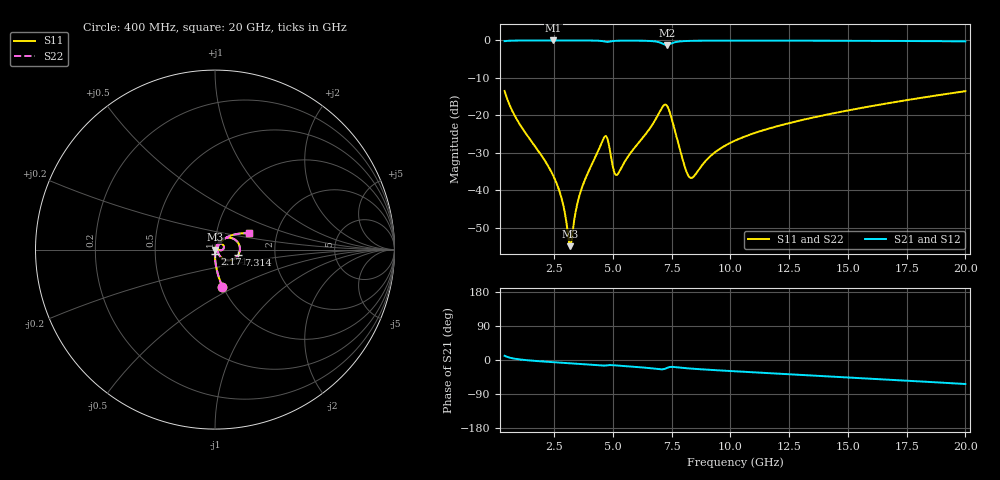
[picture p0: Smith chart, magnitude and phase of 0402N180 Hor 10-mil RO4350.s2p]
# GHz S MA R 50
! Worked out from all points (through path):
!   1960 points, 400 MHz to 20 GHz, reference 50 ohm
!   highest |S21| = -0.01 dB at 2.471 GHz (marker M1); lowest = -1.2 dB at 7.294 GHz (marker M2)
!   group delay of S21, straight-line fit = 9.13 ps
!   lowest |S11| = -54.9 dB at 3.191 GHz (marker M3), VSWR 1.00, Z = 50.2 - j0.0248 ohm
!   |S11| at or under -10 dB: start of sweep to end of sweep
!   |S22| runs from -54.9 to -13.5 dB; largest |S21 - S12| = 0
!   S11 on the Smith chart (normalised r, x): 400 MHz: 0.99, -0.43; 2.171 GHz: 1.00, -0.05; 7.314 GHz: 1.30, -0.08; 20 GHz: 1.44, +0.27
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0.4  0.2115 -78.7  0.9766 11.1  0.9766 11.1  0.2115 -78.7
0.9602859  0.08376 -87.1  0.9954 2.2  0.9954 2.2  0.08376 -87.1
2.170904  0.0232 -91.2  0.9983 -4.6  0.9983 -4.6  0.0232 -91.2
2.471057  0.01559 -90.4  0.9983 -5.8  0.9983 -5.8  0.01559 -90.4
2.83124  0.007625 -85.1  0.9982 -7.2  0.9982 -7.2  0.007625 -85.1
3.191424  0.001794 -7.9  0.9981 -8.6  0.9981 -8.6  0.001794 -7.9
3.471567  0.006166 60.9  0.9978 -9.7  0.9978 -9.7  0.006166 60.9
3.671669  0.01043 66.5  0.9974 -10.5  0.9974 -10.5  0.01043 66.5
4.642164  0.05129 35.7  0.9664 -14.8  0.9664 -14.8  0.05129 35.7
4.772231  0.04879 8.3  0.9545 -13.9  0.9545 -13.9  0.04879 8.3
5.042369  0.01837 3.1  0.9822 -13.9  0.9822 -13.9  0.01837 3.1
5.18244  0.0161 29.4  0.9881 -14.6  0.9881 -14.6  0.0161 29.4
6.943338  0.1037 39.9  0.9497 -24.0  0.9497 -24.0  0.1037 39.9
7.293517  0.1357 -8.9  0.8667 -21.3  0.8667 -21.3  0.1357 -8.9
7.313527  0.1332 -12.7  0.8677 -20.7  0.8677 -20.7  0.1332 -12.7
8.073915  0.02015 -37.4  0.9803 -21.3  0.9803 -21.3  0.02015 -37.4
8.304033  0.01466 -4.4  0.9857 -22.5  0.9857 -22.5  0.01466 -4.4
9.274528  0.03078 50.5  0.9922 -26.5  0.9922 -26.5  0.03078 50.5
10.205  0.04603 53.5  0.9932 -29.8  0.9932 -29.8  0.04603 53.5
13.46667  0.09264 46.5  0.9908 -40.8  0.9908 -40.8  0.09264 46.5
16.73834  0.1455 36.3  0.9842 -51.9  0.9842 -51.9  0.1455 36.3
20  0.2101 25.3  0.972 -63.4  0.972 -63.4  0.2101 25.3
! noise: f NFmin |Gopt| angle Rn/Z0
0.4  0.001436  0.8094  1.363  0.00157
2.571  0.005124  0.6815  7.017  0.003103
4.752  0.03837  0.9111  12.83  0.09383
6.933  0.04558  0.8928  18.61  0.09025
9.104  0.0212  0.727  24.27  0.01477
11.29  0.0188  0.6423  29.63  0.00932
13.47  0.01977  0.6089  34.83  0.008574
15.64  0.02135  0.5917  39.84  0.008544
17.82  0.02316  0.5825  44.67  0.008749
20  0.02509  0.5785  49.31  0.00907
